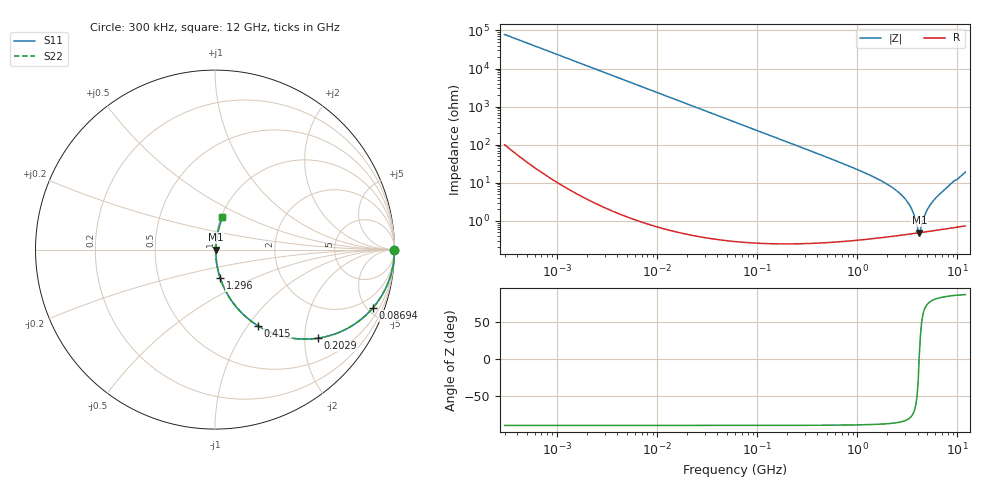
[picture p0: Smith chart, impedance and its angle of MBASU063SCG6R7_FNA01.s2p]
! MBASU063SCG6R7_FNA01  S-PARAMETER MODEL  ( General Type )
! Model Generated by TAIYO YUDEN Corporation (http://www.ty-top.com)
! Version 1.0
! TAIYO YUDEN Control No. 130801
! Copyright(c) 2013 TAIYO YUDEN CO.,LTD. All Rights Reserved.
! Product Description (link to TY-COMPAS)
! https://ds.yuden.co.jp/TYCOMPAS/or/detail?pn=MBASU063SCG6R7DFNA01&u=M
! Products Name : Multilayer Ceramic Capacitors
! Characteristics :
!  Capacitance : 6.7 pF , Rated Voltage : 50V , TCC : CG / C0G
!  Case Size : 0.6 x 0.3 / 0.024 x 0.012 [mm/inch] , Thickness : 0.3 / 0.012 [mm/inch]
!  (Conditions: Temperature = 25 degC , DC Bias Current/Voltage = 0A / 0V)
! External Node Assignments :
!  1  o---| |---o  2
! GND o---------o GND
! Frequency Range : 0.3MHz  -  12000MHz  [ 401 STEP ]
# MHz S RI R 50
! Freq[MHz].  S11 Real  S11 Imag  S21 Real  S21 Imag  S12 Real  S12 Imag  S22 Real  S22 Imag
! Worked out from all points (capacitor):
!   401 points, 300 kHz to 12 GHz, reference 50 ohm
!   read as one part in series: C = 6.75 pF near 316.3 kHz
!   lowest |Z| = 488 mohm at 4.159 GHz (marker M1)
!   series resonance near 4.142 GHz, so ESL is about 220 pH
!   S11 on the Smith chart (normalised r, x): 300 kHz: open; 86.94 MHz: 1.01, -5.42; 202.9 MHz: 1.00, -2.32; 415 MHz: 1.01, -1.12; 1.296 GHz: 1.01, -0.33; 12 GHz: 1.01, +0.38
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0.3  1 -0.00127  3.23e-06 0.00127  3.23e-06 0.00127  1 -0.00127
1.769972  0.9999 -0.00751  5.88e-05 0.00751  5.88e-05 0.00751  0.9999 -0.00751
10.44266  0.998 -0.0442  0.00197 0.0442  0.00197 0.0442  0.998 -0.0442
27.10171  0.9869 -0.1135  0.0131 0.1135  0.0131 0.1135  0.9869 -0.1135
60  0.939 -0.239  0.061 0.239  0.061 0.239  0.939 -0.239
86.94074  0.8799 -0.3246  0.1201 0.3246  0.1201 0.3246  0.8799 -0.3246
202.9496  0.5729 -0.4936  0.4271 0.4936  0.4271 0.4936  0.5729 -0.4936
353.9943  0.3047 -0.4584  0.6953 0.4584  0.6953 0.4584  0.3047 -0.4584
414.98  0.2412 -0.4255  0.7588 0.4255  0.7588 0.4255  0.2412 -0.4255
686.4755  0.1024 -0.2989  0.8976 0.2989  0.8976 0.2989  0.1024 -0.2989
1296.429  0.0293 -0.1587  0.9707 0.1587  0.9707 0.1587  0.0293 -0.1587
2088.533  0.0108 -0.0831  0.9892 0.0831  0.9892 0.0831  0.0108 -0.0831
2650.866  0.00685 -0.0521  0.9932 0.0521  0.9932 0.0521  0.00685 -0.0521
3190.978  0.00529 -0.0299  0.9947 0.0299  0.9947 0.0299  0.00529 -0.0299
3547.679  0.00488 -0.0178  0.9951 0.0178  0.9951 0.0178  0.00488 -0.0178
3944.255  0.00477 -0.00577  0.9952 0.00577  0.9952 0.00577  0.00477 -0.00577
4158.869  0.00483 0.000526  0.9952 -0.000526  0.9952 -0.000526  0.00483 0.000526
4385.161  0.00496 0.00584  0.995 -0.00584  0.995 -0.00584  0.00496 0.00584
5006.236  0.00554 0.019  0.9945 -0.019  0.9945 -0.019  0.00554 0.019
5715.274  0.00651 0.0325  0.9935 -0.0325  0.9935 -0.0325  0.00651 0.0325
8732.115  0.0156 0.0951  0.9844 -0.0951  0.9844 -0.0951  0.0156 0.0951
12000  0.0412 0.1804  0.9588 -0.1804  0.9588 -0.1804  0.0412 0.1804
